// TwinCAT 3 PLC project Untitled1
// ProgramVersion: 3.1.4024.0
// libraries:
//   Tc2_EtherCAT, * (Beckhoff Automation GmbH)
//   Tc2_MC2, * (Beckhoff Automation GmbH)
//   Tc2_MC2_Drive, * (Beckhoff Automation GmbH)
//   Tc2_MC2_XFC, * (Beckhoff Automation GmbH)
//   Tc2_Standard, * (Beckhoff Automation GmbH)
//   Tc2_System, * (Beckhoff Automation GmbH)
//   Tc3_Module, * (Beckhoff Automation GmbH)
// project tree:
//   / GlobalTextList.TcGTLO, PlcTask.TcTTO, Visualization Manager.TcVMO
//   POUs/ MAIN.TcPOU
//   VISUs/ Visualization.TcVIS
// real-time tasks:
//   TASK PlcTask: cycle T#10ms, priority 20, ADS port 350
// motion (NC):
//   TASK NC-Task 1 SAF: cycle T#2ms, priority 4, ADS port 501
//   TASK NC-Task 1 SVB: cycle T#10ms, priority 8, ADS port 511
//   AXIS Axis 7 (id 7)
//     OtherSettings: AllowMotionCmdToSlave=true
//     encoder EncType=8
//       EncPara: ScaleFactorNumerator=360, ScaleFactorDenominator=1048576, MaxCount=#xffffffff
//     drive DrvType=9
//       DrvPara: MaxCount=#xffffffff, DriveControlDWord=#x00030100
//         Analog: VeloScale=6, TorqueSetpointScale=10, ScaleFactorActTorque=0.1
//         TimeComp: TaskDelayCycles=1
//     controller CtrType=1
//       CtrPara: PriorControlFactor=1
//         Observer: BandWidth=20
//   AXIS Axis 8 (id 8)
//     OtherSettings: AllowMotionCmdToSlave=true
//     encoder EncType=8
//       EncPara: ScaleFactorNumerator=360, ScaleFactorDenominator=1048576, MaxCount=#xffffffff
//     drive DrvType=9
//       DrvPara: MaxCount=#xffffffff, DriveControlDWord=#x00030100
//         Analog: VeloScale=6, TorqueSetpointScale=10, ScaleFactorActTorque=0.1
//         TimeComp: TaskDelayCycles=1
//     controller CtrType=1
//       CtrPara: PriorControlFactor=1
//         Observer: BandWidth=20
// I/O:
//   DEVICE Device 2 (EtherCAT) (disabled), AmsNetId 5.21.176.14.3.1
//     Drive 1 (AX5206-0000-0213) [AX5206-0000-0213 EtherCAT Drive (SoE, 2 Ch.)]
//     Drive 2 (AX5206-0000-0214) [AX5206-0000-0214 EtherCAT Drive (SoE, 2 Ch.)] (disabled)
//     Drive 3 (AX5206-0000-0213) [AX5206-0000-0213 EtherCAT Drive (SoE, 2 Ch.)] (disabled)
//   DEVICE Device 1 (EtherCAT), AmsNetId 5.21.176.14.2.1
//     Term 1 (EK1200) [EK1200-5000 EtherCAT Power supply (2A E-Bus)]
//       Term 5 (EL1202) [EL1202 2Ch. Fast Dig. Input 24V, 1µs]
//       Term 6 (EL1004) [EL1004 4Ch. Dig. Input 24V, 3ms]
//       Term 7 (EL2008) [EL2008 8Ch. Dig. Output 24V, 0.5A]
//       Term 8 (EL2032) [EL2032 2Ch. Dig. Output 24V, 2A Diag]
//       Term 9 (EK1110) [EK1110 EtherCAT extension]
//     Drive 10 (AX5206-0000-0214) [AX5206-0000-0214 EtherCAT Drive (SoE, 2 Ch.)]
// variable links:
//   (this object) <-> Device 1 (EtherCAT)/Drive 10 (AX5206-0000-0214)
//     Drive/Inputs/In/nDataIn1 <-> AT 1/Following distance
//     Drive/Inputs/In/nDataIn1 <-> AT 2/Following distance
//     Drive/Inputs/In/nDcOutputTime <-> InfoData/DcOutputShift
//     Drive/Inputs/In/nState1 <-> AT 1/Drive status word @bit 8
//     Drive/Inputs/In/nState1 <-> AT 2/Drive status word @bit 8
//     Drive/Inputs/In/nState2 <-> AT 1/Drive status word
//     Drive/Inputs/In/nState2 <-> AT 2/Drive status word
//     Drive/Inputs/In/nState4 @bit 1 <-> WcState/InputToggle
//     Drive/Inputs/In/nState4 <-> WcState/WcState
//     Drive/Outputs/Out/nCtrl1 <-> MDT 1/Master control word @bit 8
//     Drive/Outputs/Out/nCtrl1 <-> MDT 2/Master control word @bit 8
//     Drive/Outputs/Out/nDataOut1 <-> MDT 1/Position command value
//     Drive/Outputs/Out/nDataOut1 <-> MDT 2/Position command value
//     Enc/Inputs/In/nDataIn1 <-> AT 1/Position feedback 1 value
//     Enc/Inputs/In/nDataIn1 <-> AT 2/Position feedback 1 value
//     Enc/Inputs/In/nDataIn3 <-> AT 1/Probe value 1 positive edge
//     Enc/Inputs/In/nDataIn3 <-> AT 2/Probe value 1 positive edge
//     Enc/Inputs/In/nDcInputTime <-> InfoData/DcInputShift
//     Enc/Inputs/In/nState4 @bit 1 <-> WcState/InputToggle
//     Enc/Inputs/In/nState4 <-> WcState/WcState
//     Enc/Inputs/In/nState5 <-> AT 1/Probe 1 positive latched
//     Enc/Inputs/In/nState5 <-> AT 2/Probe 1 positive latched
//     Enc/Outputs/Out/nCtrl5 <-> MDT 1/Probe 1 enable
//     Enc/Outputs/Out/nCtrl5 <-> MDT 2/Probe 1 enable
//   Untitled1 Instance <-> Device 1 (EtherCAT)/Drive 10 (AX5206-0000-0214)
//     PlcTask Inputs/MAIN.Di <-> AT 1/Digital inputs, state
//     PlcTask Inputs/MAIN.axis_a_Dctime <-> AT 1/Probe 1 time positive edge
//   Untitled1 Instance <-> NC-Task 1 SAF/Axes/Axis 7
//     PlcTask Inputs/MAIN.Axis_A.NcToPlc <-> Outputs/ToPlc
//     PlcTask Outputs/MAIN.Axis_A.PlcToNc <-> Inputs/FromPlc
//   Untitled1 Instance <-> NC-Task 1 SAF/Axes/Axis 8
//     PlcTask Inputs/MAIN.Axis_B.NcToPlc <-> Outputs/ToPlc
//     PlcTask Outputs/MAIN.Axis_B.PlcToNc <-> Inputs/FromPlc

CONFIGURATION Untitled1
    RESOURCE PLC ON TwinCAT3
        TASK PlcTask(INTERVAL := T#10ms, PRIORITY := 20);
        PROGRAM MAIN WITH PlcTask : MAIN;
    END_RESOURCE
END_CONFIGURATION

// ---- POUs/MAIN.TcPOU
PROGRAM MAIN
VAR
	Axis_A: axis_ref;
	Axis_B: axis_ref;
	
	axis_a_Dctime AT %I*:t_dctime32;
	Di AT %I*:INT;
	SignalTrig:Tc2_Standard.R_TRIG;
	
	
	MC_TouchProbe1: MC_TouchProbe;//A轴 touchprobe
	MC_TouchProbe2: MC_TouchProbe;//B轴 touchprobe
	MC_AbortTrigger1: MC_AbortTrigger;
	
	XFCPositionAtTime1:XFC_PositionAtTime;
	ConvertDcTimeToPos1:ConvertDcTimeToPos;

	TriggerInput	: TRIGGER_REF; 		(* Reference to the trigger signal source. *)
	TriggerInput2: TRIGGER_REF;
	
	bAbort: BOOL;

	bLatch: BOOL;
	MC_Power1: MC_Power;
	MC_MoveVelocity1: MC_MoveVelocity;
	bMove: BOOL;
	ENABLE: BOOL;
	Ready: BOOL;
	MC_Stop1: MC_Stop;
	bStop: BOOL;
	MC_Reset1: MC_Reset;
	bReset: BOOL;
	SoEReset1: FB_SoEReset;

	Trigactpos: LREAL; //上升沿获取到的位置
	Axis_A_TouchRecordedPos: LREAL;
	Axis_B_TouchRecordedPos: LREAL;//touchprobe获取到的B轴位置

	Axis_B_DctimePos: LREAL;
	Axis_B_XFCDctimePos: LREAL;
	DcTimeDiff: LREAL;
	
	Touch_ActposDiff: LREAL;
	Dcpos_ActposDiff: LREAL;
	Touch_DcposDiff: LREAL;	
END_VAR

Motion();
Axis_A.ReadStatus();
TriggerInput.EncoderID:=Axis_A.NcToPlc.AxisId;
TriggerInput2.EncoderID:=Axis_B.NcToPlc.AxisId;
TouchProbe();

IF MC_TouchProbe1.Done THEN
bLatch:=FALSE;
XFCPositionAtTime1(
	DcTime:= axis_a_Dctime, 
	Options:= , 
	Position=>Axis_B_XFCDctimePos , 
	Error=> , 
	ErrorID=> , 
	Axis:=Axis_B );
ConvertDcTimeToPos1(
	nAxisId:=Axis_B.NcToPlc.AxisId , 
	nSubIdx:=0 , 
	dcTime:=axis_a_Dctime , 
	fPosition=>Axis_B_DctimePos , 
	iErr=> );

END_IF
	
SignalTrig(CLK:= Di.1 , Q=> );
IF SignalTrig.Q THEN
		Trigactpos:=Axis_B.NcToPlc.ActPos;
END_IF

DcTimeDiff:=	Axis_B_XFCDctimePos - Axis_B_DctimePos;

Touch_ActposDiff:=Axis_B_TouchRecordedPos - Trigactpos;
Dcpos_ActposDiff:=Axis_B_XFCDctimePos - Trigactpos;
Touch_DcposDiff:=Axis_B_TouchRecordedPos - Axis_B_XFCDctimePos;

ACTION motion:
MC_Power1(
	Axis:=Axis_A, 
	Enable:=1, 
	Enable_Positive:= 1, 
	Enable_Negative:=1 , 
	Override:= , 
	BufferMode:= , 
	Options:= , 
	Status=> , 
	Busy=> , 
	Active=> , 
	Error=> , 
	ErrorID=> );
	
MC_Power1(
	Axis:=Axis_B , 
	Enable:=1, 
	Enable_Positive:= 1, 
	Enable_Negative:=1 , 
	Override:= , 
	BufferMode:= , 
	Options:= , 
	Status=> , 
	Busy=> , 
	Active=> , 
	Error=> , 
	ErrorID=> );
	

MC_MoveVelocity1(
	Axis:=Axis_B  , 
	Execute:=bMove , 
	Velocity:=360*5 , 
	Acceleration:= , 
	Deceleration:= , 
	Jerk:= , 
	Direction:= , 
	BufferMode:= , 
	Options:= , 
	InVelocity=> , 
	Busy=> , 
	Active=> , 
	CommandAborted=> , 
	Error=> , 
	ErrorID=> );	
	
	
	
MC_Reset1(
	Axis:=Axis_A , 
	Execute:=bReset , 
	Done=> , 
	Busy=> , 
	Error=> , 
	ErrorID=> );
END_ACTION

ACTION TouchProbe:
MC_TouchProbe1(
	Axis:= Axis_A, 
	TriggerInput:=TriggerInput , 
	Execute:= bLatch, 
	WindowOnly:= , 
	FirstPosition:= , 
	LastPosition:= , 
	Done=> , 
	Busy=> , 
	CommandAborted=> , 
	Error=> , 
	ErrorID=> , 
	RecordedPosition=> Axis_A_TouchRecordedPos, 
	RecordedData=> );
MC_TouchProbe2(
	Axis:= Axis_B, 
	TriggerInput:=TriggerInput2 , 
	Execute:= bLatch, 
	WindowOnly:= , 
	FirstPosition:= , 
	LastPosition:= , 
	Done=> , 
	Busy=> , 
	CommandAborted=> , 
	Error=> , 
	ErrorID=> , 
	RecordedPosition=> Axis_B_TouchRecordedPos, 
	RecordedData=> );
	
	
MC_AbortTrigger1(
	Axis:=Axis_A , 
	TriggerInput:= TriggerInput, 
	Execute:= bAbort, 
	Done=> , 
	Busy=> , 
	Error=> , 
	ErrorID=> );
END_ACTION

END_PROGRAM

// ---- VISUs/Visualization.TcVIS
VISUALIZATION Visualization  // 2x2
END_VISUALIZATION
